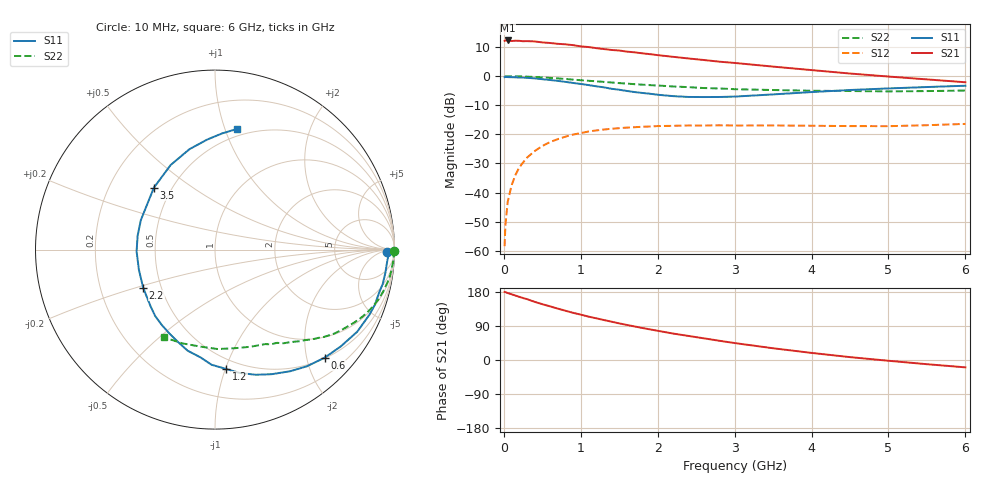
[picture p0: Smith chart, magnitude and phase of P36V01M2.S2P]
! SIEMENS Small Signal Semiconductors
! BFP181
! Si NPN RF Bipolar Junction Transistor in SOT143
! VCE = 6 V  IC = 1.2 mA
! Common Emitter S-Parameters:  March  1996
# GHz  S  MA  R  50
!  f  S11  S21  S12  S22
! GHz  MAG  ANG  MAG  ANG  MAG  ANG  MAG  ANG
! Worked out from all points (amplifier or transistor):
!   36 points, 10 MHz to 6 GHz, reference 50 ohm
!   highest |S21| = 12.2 dB at 50 MHz (marker M1)
!   |S21| within 3 dB of that: start of sweep to 1.316 GHz
!   unconditionally stable (mu >= 1): 2.982 GHz to end of sweep
!   at 250 MHz: K = 0.10, MSG = 20.8 dB, |S12| = -29.7 dB
!   at 1.4 GHz: K = 0.52, MSG = 13.5 dB, |S12| = -18.1 dB
!   at 6 GHz: K = 1.24, MAG = 4.2 dB, |S12| = -16.4 dB
!   S11 on the Smith chart (normalised r, x): 10 MHz: 44, -15; 600 MHz: 0.52, -2.35; 1.2 GHz: 0.42, -1.01; 2.2 GHz: 0.40, -0.21; 3.5 GHz: 0.40, +0.36; 6 GHz: 0.44, +1.10
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0.01  0.9605 -0.8  4.039 179.5  0.0012 82.1  0.9991 -0.3
0.02  0.9681 -1.6  4.094 179.2  0.0027 87.1  0.9948 -0.7
0.05  0.9618 -3.8  4.096 176.7  0.0069 90.1  0.9963 -1.9
0.1  0.958 -7.8  4.007 173.5  0.0132 83.7  0.9954 -3.6
0.2  0.9445 -15.2  4.033 166.7  0.0269 80.4  0.9892 -7.2
0.4  0.915 -30.0  3.942 153.5  0.0515 70.4  0.9659 -14.0
0.6  0.858 -44.5  3.706 141.6  0.0736 61.4  0.9329 -20.2
0.8  0.7966 -58.3  3.519 130.0  0.0911 53.5  0.8927 -25.7
0.9  0.7628 -65.5  3.401 124.5  0.099 49.4  0.8701 -28.3
1.1  0.7015 -78.6  3.157 114.5  0.1118 42.6  0.8318 -32.8
1.2  0.6681 -84.6  3.024 110.1  0.1167 39.4  0.8142 -35.0
1.5  0.5836 -105.1  2.75 96.6  0.1277 31.9  0.7583 -40.4
1.7  0.5321 -118.5  2.558 88.5  0.1326 27.4  0.7266 -43.7
1.9  0.498 -132.0  2.382 80.8  0.1364 23.4  0.6998 -46.7
2.2  0.4531 -152.1  2.145 69.8  0.1401 18.8  0.6643 -50.9
2.8  0.438 170.0  1.771 50.8  0.143 11.4  0.6135 -59.3
3  0.4448 158.2  1.684 44.7  0.1417 9.6  0.5958 -62.1
3.5  0.485 134.5  1.456 31.0  0.1421 6.1  0.5769 -69.7
4  0.532 117.7  1.269 18.7  0.1404 3.7  0.5605 -78.6
4.5  0.5772 104.3  1.107 7.6  0.1386 2.0  0.5542 -88.5
5.5  0.6491 86.4  0.878 -11.1  0.1435 3.9  0.5531 -109.2
6  0.6836 79.6  0.784 -19.4  0.1511 3.8  0.565 -120.0
